FUNCTION_BLOCK FB_GET_MIN_MAX
VAR CONSTANT
   // Counter initialization dependent by
   // lowest input frequency 1/(2*f*cyclTime)
   // used during offset adjust
   CMMcnt :UINT := 200;
END_VAR
VAR_INPUT
   bInit :BOOL := TRUE;
   nInputValue :DINT;END_VAR
VAR_OUTPUT
   bRESULT :BOOL;
   nMaxVal :DINT :=0;
   nMinVal :DINT :=0;
END_VAR
VAR
   nMaxValCnt :UINT;
   nMinValCnt :UINT;
   bValidMinVal :BOOL;
   bValidMaxVal :BOOL;
END_VAR

IF bInit THEN
   nMaxValCnt :=CMMcnt;
   nMinValCnt :=CMMcnt;
   nMaxVal := 0;
   nMinVal := 0;
   bInit := FALSE;
END_IF
// Assertions: new min/max values exists:
bValidMaxVal := TRUE;
bValidMinVal := TRUE;
// Filter min/max values
IF nMaxVal < nInputValue THEN
   bValidMaxVal := FALSE;
   nMaxVal := nInputValue; // Max value was found
END_IF
IF nMinVal > nInputValue THEN
   bValidMinVal := FALSE;
   nMinVal := nInputValue; // Min value was found
END_IF
// Count down, if no new value come in:
IF bValidMaxVal AND nMaxValCnt > 0 THEN
   nMaxValCnt := nMaxValCnt - 1;
END_IF
// Count down, if no new value come in:
IF bValidMinVal AND nMinValCnt > 0 THEN
   nMinValCnt := nMinValCnt - 1;
END_IF
IF ((nMaxValCnt = 0) AND (nMinValCnt = 0)) THEN
   // Consequence: min/max determined
   bInit := TRUE; // Prepare next call
   bRESULT := TRUE; // Sign valid results
ELSE
   bRESULT := FALSE; // Sign still invalid results
END_IF

END_FUNCTION_BLOCK
